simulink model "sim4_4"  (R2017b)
settings: Solver=ode4  StartTime=0.0  StopTime=50  FixedStep=0.001  RelTol=1e-3
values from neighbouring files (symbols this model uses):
  den = [1 2 1 0]    [task4_4.m]
  Kp = Kc*0.45    (= 0.9)    [task4_4.m]
  num = K    (= 1)    [task4_4.m]
  Ti = Tc/1.2    (= 5.23333333333)    [task4_4.m]
libraries: simulink x1

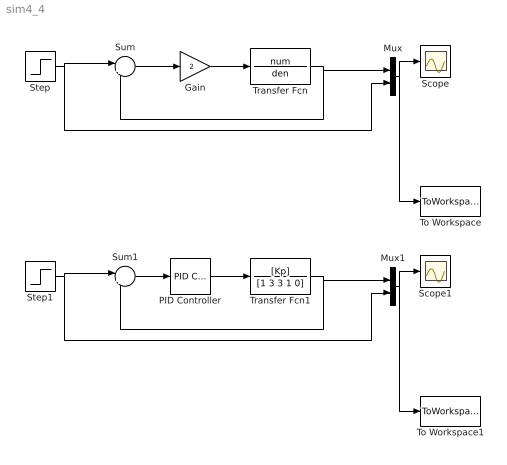
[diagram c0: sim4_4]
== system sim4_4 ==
  Gain : Gain  Gain=2
  Mux : Mux  Inputs=2
  Mux1 : Mux  Inputs=2
  PID Controller : simulink/Continuous/PID Controller  Controller=PID  TimeDomain=Continuous-time  SampleTime=-1  IntegratorMethod=Forward Euler  FilterMethod=Forward Euler  Form=Ideal  UseFilter=on  ControllerParametersSource=internal  P=Kp  I=1/Ti  D=0  N=100  InitialConditionSource=internal  InitialConditionForIntegrator=0  InitialConditionForFilter=0  ExternalReset=none  LimitOutput=off  UpperSaturationLimit=inf  LowerSaturationLimit=-inf  LinearizeAsGain=on  AntiWindupMode=none  Kb=1  TrackingMode=off  Kt=1  PParamMin=[]  PParamMax=[]  IParamMin=[]  IParamMax=[]  DParamMin=[]  DParamMax=[]  NParamMin=[]  NParamMax=[]  KbParamMin=[]  KbParamMax=[]  KtParamMin=[]  KtParamMax=[]  POutMin=[]  POutMax=[]  IOutMin=[]  IOutMax=[]  DOutMin=[]  DOutMax=[]  NOutMin=[]  NOutMax=[]  KbOutMin=[]  KbOutMax=[]  KtOutMin=[]  KtOutMax=[]  IntegratorOutMin=[]  IntegratorOutMax=[]  FilterOutMin=[]  FilterOutMax=[]  SumOutMin=[]  SumOutMax=[]  SumI1OutMin=[]  SumI1OutMax=[]  SumI2OutMin=[]  SumI2OutMax=[]  SumI3OutMin=[]  SumI3OutMax=[]  SumDOutMin=[]  SumDOutMax=[]  SaturationOutMin=[]  SaturationOutMax=[]  IntegratorContinuousStateAttributes=''  IntegratorStateMustResolveToSignalObject=off  IntegratorRTWStateStorageClass=Auto  FilterContinuousStateAttributes=''  FilterStateMustResolveToSignalObject=off  FilterRTWStateStorageClass=Auto  DifferentiatorICPrevScaledInput=0  DifferentiatorOutMin=[]  DifferentiatorOutMax=[]  InitialConditionSetting=State (most efficient)  FilterDiffOutCoefMin=[]  FilterDiffOutCoefMax=[]  SumDenOutMin=[]  SumDenOutMax=[]  SumNumOutMin=[]  SumNumOutMax=[]  ReciprocalOutMin=[]  ReciprocalOutMax=[]  DivideOutMin=[]  DivideOutMax=[]  TunerSelectOption=Transfer Function Based (PID Tuner App)
  Scope : Scope
  Scope1 : Scope
  Step : Step  Time=0  SampleTime=0
  Step1 : Step  SampleTime=0
  Sum : Sum  Inputs=|+-
  Sum1 : Sum  Inputs=|+-
  To Workspace : ToWorkspace  VariableName=simout  SaveFormat=Timeseries  SampleTime=-1
  To Workspace1 : ToWorkspace  VariableName=simout1  SaveFormat=Timeseries  SampleTime=-1
  Transfer Fcn : TransferFcn  Numerator=num  Denominator=den
  Transfer Fcn1 : TransferFcn  Numerator=[Kp]  Denominator=[1 3 3 1 0]
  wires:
  Step/1 -> Mux/2, Sum/1
  Sum/1 -> Gain/1
  Gain/1 -> Transfer Fcn/1
  Transfer Fcn/1 -> Mux/1, Sum/2
  Mux/1 -> To Workspace/1, Scope/1
  Mux1/1 -> To Workspace1/1, Scope1/1
  Sum1/1 -> PID Controller/1
  Step1/1 -> Mux1/2, Sum1/1
  Transfer Fcn1/1 -> Mux1/1, Sum1/2
  PID Controller/1 -> Transfer Fcn1/1
